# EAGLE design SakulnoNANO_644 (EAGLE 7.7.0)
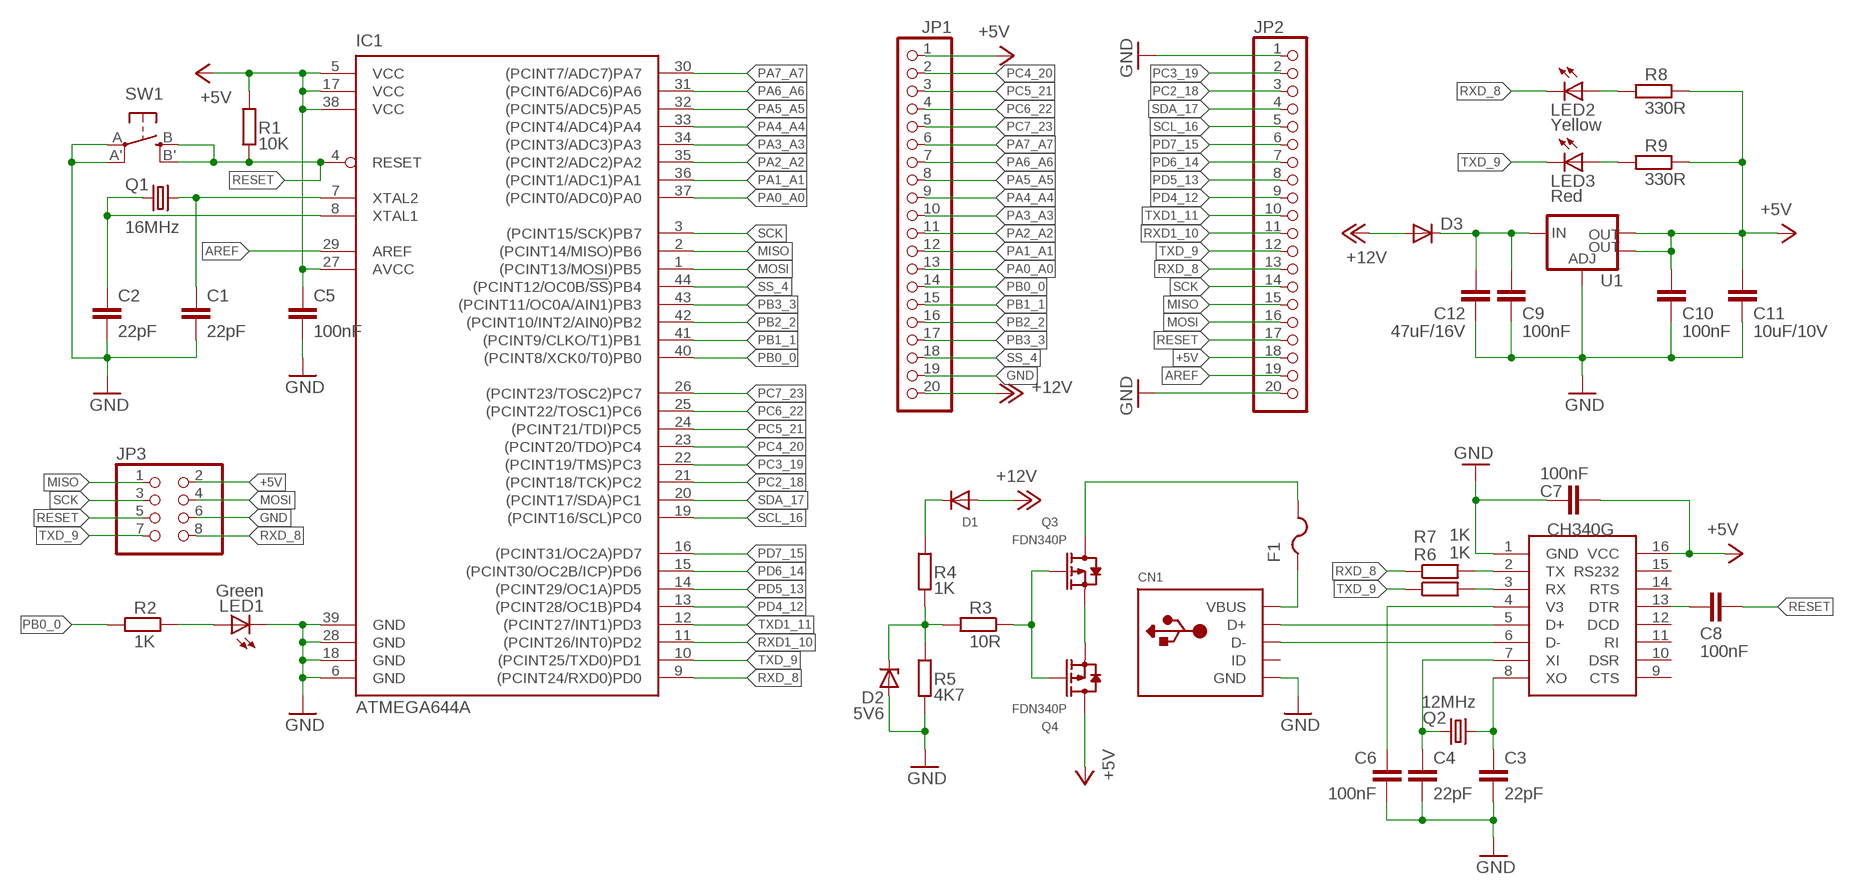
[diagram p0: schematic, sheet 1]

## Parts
C1  22pF  C-EUC1206  [C1206]
C2  22pF  C-EUC1206  [C1206]
C3  22pF  C-EUC1206  [C1206]
C4  22pF  C-EUC1206  [C1206]
C5  100nF  C-EUC1206  [C1206]
C6  100nF  C-EUC1206  [C1206]
C7  100nF  C-EUC1206  [C1206]
C8  100nF  C-EUC1206  [C1206]
C9  100nF  C-EUC1206  [C1206]
C10  100nF  C-EUC1206  [C1206]
C11  10uF/10V  C-EUC1206  [C1206]
C12  47uF/16V  C-EUC1206  [C1206]
CN1  USBMINIB  [USB-MINIB]
D1  DIODE_SOD-123FL  [SOD-123FL]
D2  5V6  ZENER-DIODESOD80C  [SOD80C]
D3  DIODE-DO214AC  [DO214AC]
F1  PTCFUSE-1206  [R1206]
IC1  ATMEGA644A  [TQFP44]
JP1  PINHD-1X20-BIG  [1X20-BIG]
JP2  PINHD-1X20-BIG  [1X20-BIG]
JP3  PINHD-2X4  [2X04]
LED1  Green  LEDCHIPLED_1206  [CHIPLED_1206]
LED2  Yellow  LEDCHIPLED_1206  [CHIPLED_1206]
LED3  Red  LEDCHIPLED_1206  [CHIPLED_1206]
Q1  16MHz  CRYSTALSM49  [SM49]
Q2  12MHz  CRYSTALSM49  [SM49]
Q3  FDN340P  SMD-MOSFET-P-CH-20V-2A-FDN340P(SOT-23)  [SOT-23]
Q4  FDN340P  SMD-MOSFET-P-CH-20V-2A-FDN340P(SOT-23)  [SOT-23]
R1  10K  R-EU_R1206  [R1206]
R2  1K  R-EU_R1206  [R1206]
R3  10R  R-EU_R1206  [R1206]
R4  1K  R-EU_R1206  [R1206]
R5  4K7  R-EU_R1206  [R1206]
R6  1K  R-EU_R1206  [R1206]
R7  1K  R-EU_R1206  [R1206]
R8  330R  R-EU_R1206  [R1206]
R9  330R  R-EU_R1206  [R1206]
SW1  SPST_TACT-EVQQ2  [EVQ-Q2]
U1  V_REG_LM1117SOT223  [SOT223]
U$1  CH340G  [SOIC16]

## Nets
+5V: C5.1 C7.2 C10.2 C11.2 IC1.5(VCC) IC1.17(VCC) IC1.27(AVCC) IC1.38(VCC) JP1.1 JP2.18 JP3.2 Q4.3(D) R1.2 R8.1 R9.1 U1.2(OUT) U1.4(OUT) U$1.16(VCC)
+12V: D1.A D3.A JP1.20
AREF: IC1.29(AREF) JP2.19
GND: C1.2 C2.2 C3.2 C4.2 C5.2 C6.2 C7.1 C9.1 C10.1 C11.1 C12.1 CN1.GND D2.A IC1.6(GND) IC1.18(GND) IC1.28(GND) IC1.39(GND) JP1.19 JP2.1 JP2.20 JP3.6 LED1.C R5.2 SW1.A'(P1) SW1.A(P) U1.1(ADJ) U$1.1(GND)
MISO: IC1.2((PCINT14/MISO)PB6) JP2.15 JP3.1
MOSI: IC1.1((PCINT13/MOSI)PB5) JP2.16 JP3.4
N$1: LED1.A R2.1
N$2: CN1.D+ U$1.5(D+)
N$3: C1.1 IC1.7(XTAL2) Q1.2
N$4: C2.1 IC1.8(XTAL1) Q1.1
N$5: CN1.D- U$1.6(D-)
N$6: CN1.VBUS F1.1
N$7: C4.1 Q2.1 U$1.7(XI)
N$8: C3.1 Q2.2 U$1.8(XO)
N$9: C8.1 U$1.13(DTR)
N$10: C6.1 U$1.4(V3)
N$11: R7.2 U$1.2(TX)
N$12: R6.2 U$1.3(RX)
N$13: Q3.2(S) Q4.2(S)
N$14: Q3.1(G) Q4.1(G) R3.1
N$15: D2.C R3.2 R4.2 R5.1
N$16: D1.C R4.1
N$17: LED2.A R8.2
N$18: LED3.A R9.2
N$22: C9.2 C12.2 D3.C U1.3(IN)
PA0_A0: IC1.37((PCINT0/ADC0)PA0) JP1.13
PA1_A1: IC1.36((PCINT1/ADC1)PA1) JP1.12
PA2_A2: IC1.35((PCINT2/ADC2)PA2) JP1.11
PA3_A3: IC1.34((PCINT3/ADC3)PA3) JP1.10
PA4_A4: IC1.33((PCINT4/ADC4)PA4) JP1.9
PA5_A5: IC1.32((PCINT5/ADC5)PA5) JP1.8
PA6_A6: IC1.31((PCINT6/ADC6)PA6) JP1.7
PA7_A7: IC1.30((PCINT7/ADC7)PA7) JP1.6
PB0_0: IC1.40((PCINT8/XCK0/T0)PB0) JP1.14 R2.2
PB1_1: IC1.41((PCINT9/CLKO/T1)PB1) JP1.15
PB2_2: IC1.42((PCINT10/INT2/AIN0)PB2) JP1.16
PB3_3: IC1.43((PCINT11/OC0A/AIN1)PB3) JP1.17
PC2_18: IC1.21((PCINT18/TCK)PC2) JP2.3
PC3_19: IC1.22((PCINT19/TMS)PC3) JP2.2
PC4_20: IC1.23((PCINT20/TDO)PC4) JP1.2
PC5_21: IC1.24((PCINT21/TDI)PC5) JP1.3
PC6_22: IC1.25((PCINT22/TOSC1)PC6) JP1.4
PC7_23: IC1.26((PCINT23/TOSC2)PC7) JP1.5
PD4_12: IC1.13((PCINT28/OC1B)PD4) JP2.9
PD5_13: IC1.14((PCINT29/OC1A)PD5) JP2.8
PD6_14: IC1.15((PCINT30/OC2B/ICP)PD6) JP2.7
PD7_15: IC1.16((PCINT31/OC2A)PD7) JP2.6
RESET: C8.2 IC1.4(RESET) JP2.17 JP3.5 R1.1 SW1.B'(S1) SW1.B(S)
RXD1_10: IC1.11((PCINT26/INT0)PD2) JP2.11
RXD_8: IC1.9((PCINT24/RXD0)PD0) JP2.13 JP3.8 LED2.C R7.1
SCK: IC1.3((PCINT15/SCK)PB7) JP2.14 JP3.3
SCL_16: IC1.19((PCINT16/SCL)PC0) JP2.5
SDA_17: IC1.20((PCINT17/SDA)PC1) JP2.4
SS_4: IC1.44((PCINT12/OC0B/!SS!)PB4) JP1.18
TXD1_11: IC1.12((PCINT27/INT1)PD3) JP2.10
TXD_9: IC1.10((PCINT25/TXD0)PD1) JP2.12 JP3.7 LED3.C R6.1
VBUS: F1.2 Q3.3(D)
Unconnected: CN1.ID U$1.9(CTS) U$1.10(DSR) U$1.11(RI) U$1.12(DCD) U$1.14(RTS) U$1.15(RS232)

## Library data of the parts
C1-C12 = rcl:C-EU: CAPACITOR, European symbol
CN1 = adafruit:USB: USB Connectors USBMINIB - Surface Mount Female Mini-B USB Connector 4UConnector: 06564 By microbuilder.eu Thru-hole RA Female Mini-B USB Connector 4UConnector: 18732 By ladyada.net
D1 = adafruit:DIODE: Diode
D2 = diode:ZENER-DIODE: Z-Diode
D3 = diode:DIODE-: DIODE
F1 = adafruit:PTCFUSE: PTC fuses, resettable thermistors
IC1 = atmel:ATMEGA644: 8-bit Microcontroller with 64K Bytes In-System Programmable Flash Source: http://www.atmel.com/dyn/resources/prod_documents/doc2593.pdf; MPN: ATMEGA644PV-10AU; OC_FARNELL: 1455123; OC_NEWARK: 58M3748
JP1 JP2 = adafruit:PINHD-1X20: PIN HEADER
JP3 = pinhead:PINHD-2X4: PIN HEADER
LED1-LED3 = adafruit:LED: LED
Q1 Q2 = crystal:CRYSTAL: CRYSTAL; OC_FARNELL: unknown; OC_NEWARK: unknown
Q3 Q4 = Seeed-Transistor:SMD-MOSFET-P-CH-20V-2A-FDN340P(SOT-23): 305030026; MPN: FDN340P
R1-R9 = rcl:R-EU_: RESISTOR, European symbol
SW1 = adafruit:SPST_TACT: SMT 6mm switch, EVQQ2 series http://www.ladyada.net/library/eagle
U1 = SparkFun-IC-Power:V_REG_LM1117: Voltage Regulator LM1117 Standard adjustable voltage regulator but in SMD form. Spark Fun Electronics SKU : COM-00595; PROD_ID: VREG-08170
U$1 = ch340g:CH340G

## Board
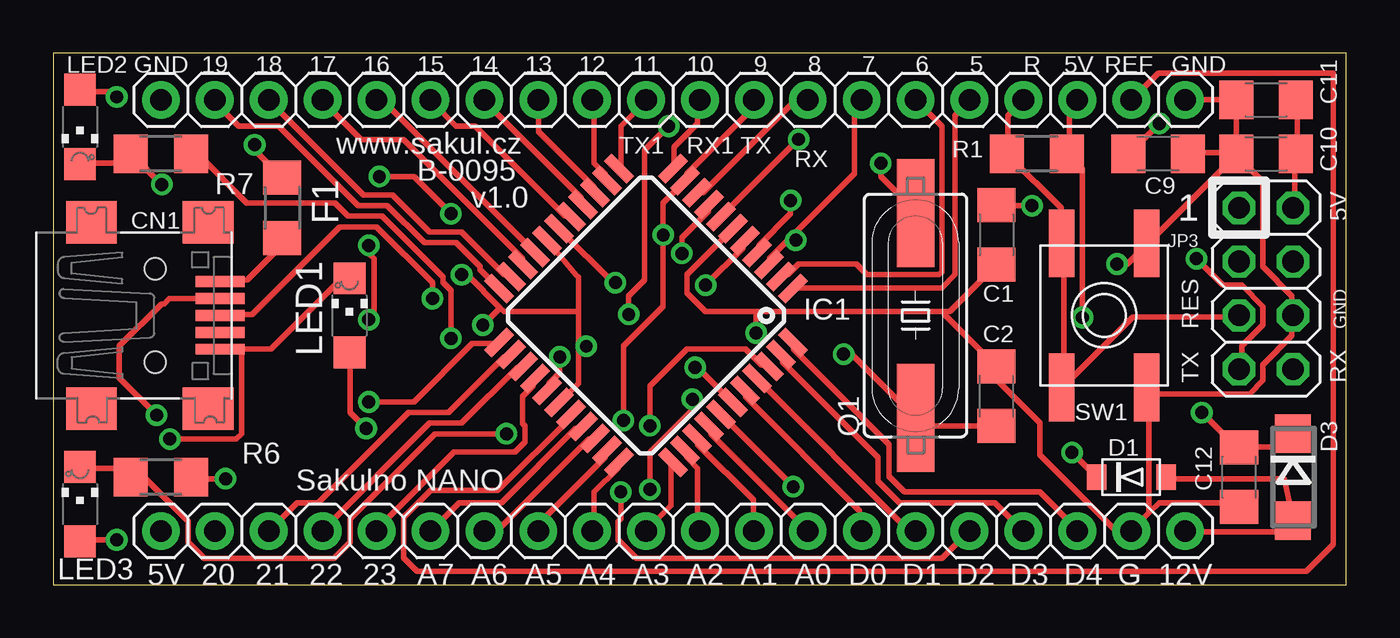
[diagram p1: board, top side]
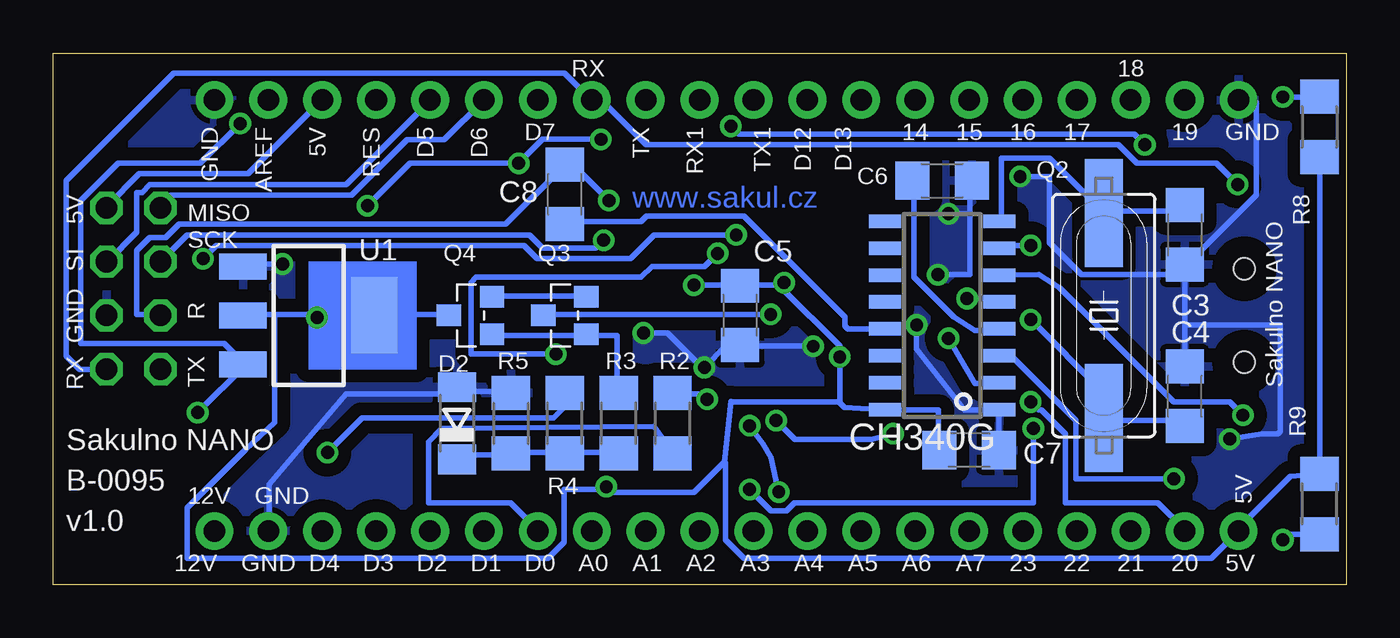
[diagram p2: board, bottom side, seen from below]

Size 60.94 x 25.07 mm. Coordinates in mm from the lower left corner, seen from the top.
Outline: 0,0 60.94,0 60.94,25.07 0,25.07 0,0
Copper layers (1*16): Top 0.035mm / dielectric 1.5mm / Bottom 0.035mm
Design rules "default": minimum track width 10mil, minimum drill 24mil, track to track 8mil, track to pad 8mil, pad to pad 8mil, via to via 8mil, smd to smd 8mil, copper to edge 40mil, drill to drill 8mil, minimum pad ring 10mil, minimum via ring 8mil, stop-mask expansion 4mil, vias tented up to drill 0mil, thermal gap 10mil

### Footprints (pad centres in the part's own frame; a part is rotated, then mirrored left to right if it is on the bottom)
C1206 = smd 1.6 x 1.8: 1 -1.4,0; 2 1.4,0
USB-MINIB = smd 0.5 x 2.308: D+ 0,4.064; D- -0.8,4.064; GND 1.6,4.064; ID 0.8,4.064; VBUS -1.6,4.064 | smd 2 x 2.4: GND1 -4.4,-2; GND2 -4.4,3.5; GND3 4.4,3.5; GND4 4.4,-2 | hole 1: -2.2,1; 2.2,1
SOD-123FL = smd 0.91 x 1.22: A 1.637,0; C -1.637,0
SOD80C = smd 1.4 x 1.8: A 1.7,0; C -1.7,0
DO214AC = smd 1.8 x 1.7: A 2.05,0; C -2.05,0
R1206 = smd 1.6 x 1.803: 1 -1.422,0; 2 1.422,0
TQFP44 = smd 1.5 x 0.5: 1 -5.8,4; 2 -5.8,3.2; 3 -5.8,2.4; 4 -5.8,1.6; 5 -5.8,0.8; 6 -5.8,0; 7 -5.8,-0.8; 8 -5.8,-1.6; 9 -5.8,-2.4; 10 -5.8,-3.2; 11 -5.8,-4; 23 5.8,-4; 24 5.8,-3.2; 25 5.8,-2.4; 26 5.8,-1.6; 27 5.8,-0.8; 28 5.8,0; 29 5.8,0.8; 30 5.8,1.6; 31 5.8,2.4; 32 5.8,3.2; 33 5.8,4 | smd 0.5 x 1.5: 12 -4,-5.8; 13 -3.2,-5.8; 14 -2.4,-5.8; 15 -1.6,-5.8; 16 -0.8,-5.8; 17 0,-5.8; 18 0.8,-5.8; 19 1.6,-5.8; 20 2.4,-5.8; 21 3.2,-5.8; 22 4,-5.8; 34 4,5.8; 35 3.2,5.8; 36 2.4,5.8; 37 1.6,5.8; 38 0.8,5.8; 39 0,5.8; 40 -0.8,5.8; 41 -1.6,5.8; 42 -2.4,5.8; 43 -3.2,5.8; 44 -4,5.8
1X20-BIG = drill 1.016 pad 1.778: 1 -24.13,0; 2 -21.59,0; 3 -19.05,0; 4 -16.51,0; 5 -13.97,0; 6 -11.43,0; 7 -8.89,0; 8 -6.35,0; 9 -3.81,0; 10 -1.27,0; 11 1.27,0; 12 3.81,0; 13 6.35,0; 14 8.89,0; 15 11.43,0; 16 13.97,0; 17 16.51,0; 18 19.05,0; 19 21.59,0; 20 24.13,0
2X04 = drill 1.016 octagon: 1 -3.81,-1.27; 2 -3.81,1.27; 3 -1.27,-1.27; 4 -1.27,1.27; 5 1.27,-1.27; 6 1.27,1.27; 7 3.81,-1.27; 8 3.81,1.27
CHIPLED_1206 = smd 1.5 x 1.5: A 0,-1.75; C 0,1.75
SM49 = smd 5.08 x 1.778: 1 -4.826,0; 2 4.826,0
SOT-23 = smd 1.016 x 1.143: 1 -0.889,-1.016; 2 0.889,-1.016; 3 0,1.016
EVQ-Q2 = smd 3.2 x 1.2: A -3.4,-2; A' 3.4,-2; B -3.4,2; B' 3.4,2
SOT223 = smd 1.219 x 2.235: 1 -2.311,-3.099; 2 0,-3.099; 3 2.311,-3.099 | smd 3.6 x 2.2: 4 0,3.099
SOIC16 = smd 0.635 x 1.524: 1 -4.445,-2.695; 2 -3.175,-2.695; 3 -1.905,-2.695; 4 -0.635,-2.695; 5 0.635,-2.695; 6 1.905,-2.695; 7 3.175,-2.695; 8 4.445,-2.695; 9 4.445,2.695; 10 3.175,2.695; 11 1.905,2.695; 12 0.635,2.695; 13 -0.635,2.695; 14 -1.905,2.695; 15 -3.175,2.695; 16 -4.445,2.695

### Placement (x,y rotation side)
C1  44.45,16.51 270 top
C2  44.45,8.89 90 top
C3  7.62,16.51 270 bottom
C4  7.62,8.89 90 bottom
C5  28.57,12.7 270 bottom
C6  19.05,19.05 0 bottom
C7  17.78,6.35 180 bottom
C8  36.83,18.41 90 bottom
C9  52.07,20.32 180 top
C10  57.15,20.32 0 top
C11  57.15,22.86 0 top
C12  55.88,5.08 90 top
CN1  3.81,12.7 270 top
D1  50.8,5.08 0 top
D2  41.91,7.62 90 bottom
D3  58.42,5.08 270 top
F1  10.79,17.78 90 top
IC1  27.94,12.7 225 top
JP1  29.21,2.54 0 top
JP2  29.21,22.86 0 top
JP3  57.15,13.97 270 top
LED1  13.97,12.7 0 top
LED2  1.27,21.59 180 top
LED3  1.27,3.81 0 top
Q1  40.64,12.7 90 top
Q2  11.43,12.7 90 bottom
Q3  36.83,12.7 90 bottom
Q4  41.27,12.7 90 bottom
R1  46.35,20.32 0 top
R2  31.75,7.62 270 bottom
R3  34.29,7.62 270 bottom
R4  36.83,7.62 270 bottom
R5  39.37,7.62 90 bottom
R6  5.08,5.08 0 top
R7  5.08,20.32 0 top
R8  1.27,21.59 90 bottom
R9  1.27,3.81 270 bottom
SW1  49.53,12.7 90 top
U1  48.9,12.7 270 bottom
U$1  19.05,12.7 90 bottom

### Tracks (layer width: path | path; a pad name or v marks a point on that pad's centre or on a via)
+5V  (via drill 0.61)
  Top 0.254: JP2.18 48.25,22.75 47.88,22.38 47.88,20.38 R1.2 47.88,20.25 48.5,19.62 v48.5,12.61 | C11.2 58.62,22.75 58.62,20.38 C10.2 58.5,20.25 58.5,17.88 JP3.2 | v26.5,14.25 26.38,14.25 23.88,16.75 IC1.17 | v30.75,14.12 32.5,15.88 32.5,16.12 IC1.5 | v34.88,4.62 31.5,8 IC1.38 | v23.88,10.75 23.88,10 23.38,9.5 23.38,9.25 IC1.27
  Bottom 0.254: Q4.3 42.38,12.75 45.75,12.75 U1.4 45.88,12.75 48.5,12.75 | 48.5,12.75 50.5,12.75 | 50.5,12.75 51.88,12.75 U1.2 | JP2.18 48.38,22.75 51.75,19.38 56.88,19.38 58.38,17.88 JP3.2 | v48.5,12.61 48.5,12.75 | R8.1 1.25,20.12 1.25,5.25 R9.1 2.65,5.12 5.14,2.62 5,2.62 JP1.1 5.12,2.5 6.38,1.25 28.38,1.25 29.25,2.12 29.25,5.74 29.31,5.8 | v30.75,14.12 28.62,14.12 C5.1 28.5,14.12 26.62,14.12 v26.5,14.25 26.62,14 23.88,11.25 v23.88,10.75 23.88,8.62 23.91,8.62 | 29.31,5.8 29,8.65 29,8.62 23.91,8.62 | 29.31,5.8 30.75,4.37 34.5,4.37 v34.88,4.62 34.88,4.5 36.88,4.5 36.88,2 37.62,1.25 54.62,1.25 54.62,3.63 51.88,6.38 50.5,7.66 50.5,12.75 | 23.91,8.62 23.66,8.38 U$1.16 21.62,8.25 19.23,8.25 19.23,6.38 C7.2
+12V
  Top 0.254: D1.A 52.5,5 58.02,5 58.38,3.38 58.38,3.12 D3.A 58.25,3.12 57.62,2.5 53.38,2.5 JP1.20
AREF
  Top 0.254: IC1.29 24.4,7.89 20.95,4.45 17.78,4.45 16.51,3.17 16.51,1.27 17.14,0.64 59.05,0.64 60.33,1.91 60.33,24.13 52.07,24.13 JP2.19
GND  (via drill 0.61)
  Top 0.254: LED1.C 13.88,14.38 13.52,14.38 10.27,11.12 7.88,11.12 CN1.GND 8.88,11 8.88,7.12 8.62,6.88 v5.5,6.88 | v30.25,10.25 30.38,10.25 32,8.62 IC1.39 | 24.75,11.25 24.75,9.5 23.88,8.62 IC1.28 | 24.75,11.25 24.75,12.88 | 24.75,12.88 24.75,14.5 24.64,14.61 23.38,16.12 IC1.18 | v19.25,14.62 19.5,14.62 21.06,13.06 | 21.06,13.06 21.25,12.88 24.75,12.88 | 21.06,13.06 v20.25,12.25 | 24.75,11.25 v25.12,11.25 | v15.38,19.25 17,19.25 v18.75,17.5 | v50.12,15.12 50.62,15.12 51.5,16 SW1.A' 51.62,16.12 55.75,20.25 | C9.1 53.5,20.38 55.75,20.38 C10.1 | C10.1 C11.1 55.62,22.88 53.38,22.88 JP2.20 | 55.75,20.25 57,19 57,15 58.38,13.62 58.38,12.75 JP3.6 58.38,12.62 58.38,11.75 57,10.38 57,9.62 56.38,9 51.75,9 SW1.A 51.62,9.25 51.62,3.5 51.69,3.44 | 55.75,20.25 C10.1 | 42,12.88 42.25,12.88 44.38,15 C1.2 | 42,12.88 33.12,12.88 | 33.12,12.88 30.75,12.88 29.88,13.75 29.88,14.62 32,16.75 IC1.6 | 42,12.88 42,12.75 44.38,10.38 C2.2 44.5,10.25 44.5,9.62 46.5,7.62 46.5,6.12 50,2.62 50.75,2.62 JP1.19 50.88,2.62 51.69,3.44 | 51.69,3.44 52.12,3.88 55.66,3.88 55.78,3.75 55.88,3.75 C12.1 | 33.12,12.88 v33.12,11.88
  Bottom 0.254: 7.62,12.25 7.62,15 C3.2 | 7.62,12.25 7.62,10.38 C4.2 | C3.2 7.5,15.12 4.25,18.38 4.25,22.75 5,22.75 JP2.1 | v5.5,6.88 3.98,7.12 3.23,7.12 3.12,7.23 3.12,12.25 7.62,12.25 | C7.1 16.36,6.38 16.38,6.38 16.38,8.25 U$1.1 16.5,8.25 17.12,8.24 18.01,8.24 20.25,11.12 v20.25,12.25 | 17.75,17.5 17.75,14.62 v19.25,14.62 | 17.75,17.5 17.75,19 C6.2 | v25.12,11.25 28.5,11.25 C5.2 28.62,11.25 29.25,11.25 v30.25,10.25 30.38,10.25 32,11.88 v33.12,11.88 | v15.38,19.25 14,19.25 14,16.12 12.5,14.62 7.75,14.62 C3.2 | 17.75,17.5 v18.75,17.5 | v50.12,15.12 51.88,15.12 U1.1 | R5.2 39.38,9.12 41.75,9.12 41.88,9.25 D2.A 42,9.25 42.88,9.01 47.12,9.01 50.75,4.75 50.75,2.62 JP1.19
  pour Bottom (isolate 0.61): 0,24.77 60.96,24.77 60.96,0 0,0
MISO
  Top 0.254: JP2.15 41.88,21.62 41.88,14.75 41.75,14.62 38.35,14.62 37.85,15.12 35.12,15.12 34.62,14.62 34.38,14.62 IC1.2
  Bottom 0.254: JP2.15 42.51,20.99 44.26,20.99 46.88,18.38 55.38,18.38 55.88,17.88 JP3.1
MOSI
  Top 0.254: IC1.1 34.88,14 41.88,14 42.5,14.62 42.5,22.12 43.12,22.75 JP2.16
  Bottom 0.254: JP3.4 58.38,15.25 57,16.62 57,18.5 56.75,18.5 56.38,18.88 47.12,18.88 43.25,22.75 JP2.16
N$1  (via drill 0.61)
  Top 0.254: v14.75,7.38 14,8.12 14,10.88 LED1.A | v28.12,4.5 28.12,6.25 30.12,8.25 v30.12,8.75
  Bottom 0.254: v14.75,7.38 14.75,3.88 26,3.88 26.38,3.5 27.12,3.5 v28.12,4.5 | v30.12,8.75 30.38,9 31.75,9 R2.1
N$2  (via drill 0.61)
  Top 0.254: v17.88,13.5 17.88,14.25 15.25,16.88 13.5,16.88 9.38,12.75 7.88,12.75 CN1.D+
  Bottom 0.254: v17.88,13.5 16.5,13.5 16.38,13.38 U$1.5
N$3  (via drill 0.61)
  Top 0.254: v35.12,21 31.5,17.38 IC1.7 | v39,19.88 39,19.25 40.62,17.62 Q1.2 | v46.12,17.88 44.5,17.88 C1.1
  Bottom 0.254: v35.12,21 37.88,21 v39,19.88 44.12,19.88 v46.12,17.88
N$4  (via drill 0.61)
  Top 0.254: v29.62,15.62 29.62,16.38 30.88,17.62 30.88,17.88 IC1.8 | v37.25,10.88 37.62,10.88 40.62,7.88 Q1.1 40.75,7.75 41,7.5 44.38,7.5 C2.1
  Bottom 0.254: v29.62,15.62 30.25,15 32.73,15 33.23,14.5 41,14.5 41.25,14.25 41.25,10.88 v37.25,10.88
N$5  (via drill 0.61)
  Top 0.254: v4.88,8 3.12,9.75 3.12,11.25 5.12,13.25 5.23,13.25 5.48,13.5 CN1.D-
  Bottom 0.254: U$1.6 14.48,14.63 13.5,14 8.12,8.62 5.5,8.62 v4.88,8
N$6
  Top 0.254: F1.1 10.75,16.25 11.02,16.25 9.14,14.38 CN1.VBUS
N$7  (via drill 0.61)
  Top 0.254: v14.88,16 14.88,15.62 15.12,15.38 15.12,12.75 v14.88,12.5
  Bottom 0.254: v14.88,16 16.12,16 16.25,15.88 U$1.7 | v14.88,12.5 11.5,9.12 11.5,7.88 Q2.1 11.38,7.75 7.88,7.75 C4.1
N$8
  Bottom 0.254: U$1.8 16.25,17.25 16.25,20.12 14,20.12 11.5,17.62 Q2.2 11.38,17.62 7.88,17.62 7.62,17.88 C3.1
N$9
  Bottom 0.254: C8.1 36.75,17.12 33.23,17.12 32.98,17.38 28.38,17.38 23.62,12.62 23.62,12.2 23.5,12.06 U$1.13
N$10
  Bottom 0.254: C6.1 20.38,19 20.38,14.5 18.5,12.62 17.51,11.99 16.43,11.99 U$1.4
N$11  (via drill 0.61)
  Top 0.254: v18.75,11.62 18.75,13.88 18.38,14.25 18.38,14.5 15.5,17.38 13.9,17.38 13.28,18 9.12,18 6.88,20.25 6.62,20.25 R7.2
  Bottom 0.254: v18.75,11.62 17.89,10.12 17.51,9.49 16.39,9.49 U$1.2 17.01,9.62
N$12  (via drill 0.61)
  Top 0.254: v8.12,5 6.62,5 R6.2
  Bottom 0.254: v8.12,5 12.75,5 12.75,7.75 15.88,10.88 16.39,10.88 16.25,10.75 U$1.3
N$13
  Bottom 0.254: Q3.2 35.88,13.62 40.25,13.62 Q4.2
N$14
  Bottom 0.254: Q4.1 40.25,11.75 35.88,11.75 Q3.1 35.75,11.75 34.38,11.75 34.38,9.12 R3.1
N$15
  Bottom 0.254: R3.2 34.38,6.25 36.75,6.25 R4.2 36.88,6.25 39.25,6.25 R5.1 39.38,6.12 41.75,6.12 41.88,6 D2.C
N$16  (via drill 0.61)
  Top 0.254: v48.01,6.24 49.12,5.12 D1.C
  Bottom 0.254: v48.01,6.24 46.38,7.88 37.37,7.88 36.24,9 R4.1
N$17  (via drill 0.61)
  Top 0.254: v3,23 2.75,23.25 1.38,23.25 LED2.A
  Bottom 0.254: v3,23 1.38,23 R8.2
N$18  (via drill 0.61)
  Top 0.254: v3,2.12 1.38,2.12 LED3.A
  Bottom 0.254: v3,2.12 2.75,2.38 1.38,2.38 R9.2
N$22  (via drill 0.61)
  Top 0.254: D3.C 58.38,7.12 57.75,6.5 56,6.5 C12.2 55.75,6.5 v54.12,8.12 | v52.12,21.75 50.75,20.38 C9.2
  Bottom 0.254: v52.12,21.75 54,19.88 57.88,19.88 59.62,18.12 59.62,11.38 52.88,11.38 52,10.5 U1.3 51.88,10.38 v54.12,8.12
PA0_A0
  Top 0.254: IC1.37 31,7.38 31,7.12 35.5,2.62 JP1.13
PA1_A1
  Top 0.254: IC1.36 30.38,6.88 30.38,6.62 33,4 33,2.62 JP1.12
PA2_A2
  Top 0.254: IC1.35 29.88,6.25 29.88,6 30.38,5.5 30.38,2.62 JP1.11
PA3_A3
  Top 0.254: IC1.34 29.12,5.75 29.12,3.75 28,2.62 JP1.10
PA4_A4
  Top 0.254: IC1.33 26.62,5.75 26.62,5.5 25.5,4.38 25.5,2.62 JP1.9
PA5_A5
  Top 0.254: IC1.32 26,6.25 26,6 22.88,2.88 22.88,2.62 JP1.8
PA6_A6
  Top 0.254: IC1.31 25.5,6.88 25.25,6.88 21,2.62 20.38,2.62 JP1.7
PA7_A7
  Top 0.254: IC1.30 24.88,7.38 24.62,7.38 21.12,3.88 19.12,3.88 17.88,2.62 JP1.6
PB0_0
  Top 0.254: IC1.40 32.62,9.12 32.62,8.88 38,3.5 38,2.62 JP1.14
  Bottom 0.254: R2.2 31.75,6.25 32.63,7.47 42.62,7.38 43.25,6.75 43.25,3.88 39.38,3.88 38.12,2.62 JP1.14
PB1_1
  Top 0.254: IC1.41 33.25,9.62 40.25,2.62 40.62,2.62 JP1.15
PB2_2  (via drill 0.61)
  Top 0.254: v28.12,7.5 28.12,9.38 29.88,11.12 32.62,11.12 33.38,10.38 33.62,10.38 IC1.42 | v26.75,4.38 26.75,3.12 26.62,3 26.62,2.12 27.5,1.25 41.88,1.25 43.12,2.5 JP1.16
  Bottom 0.254: v28.12,7.5 27.49,6.64 27.11,6.01 v26.75,4.38
PB3_3
  Top 0.254: IC1.43 34.38,10.75 34.38,10.5 38.88,6 38.88,4.88 39.88,3.88 44.38,3.88 45.62,2.62 JP1.17
PC2_18
  Top 0.254: IC1.21 21.5,14.62 21.25,14.62 19.25,16.62 17.75,16.62 16,18.38 14.62,18.38 10.25,22.75 JP2.3
PC3_19
  Top 0.254: IC1.22 21,14 20.12,14.88 20.12,15 19,16.12 17.5,16.12 15.75,17.88 14.38,17.88 10.62,21.62 8.75,21.62 7.62,22.75 JP2.2
PC4_20  (via drill 0.61)
  Top 0.254: v14.88,8.62 17,8.62 19.75,11.38 21,11.38 IC1.23
  Bottom 0.254: v14.88,8.62 14.5,8.25 14.38,8.25 13.25,7.12 13.25,3.88 8.88,3.88 7.62,2.62 JP1.2
PC5_21
  Top 0.254: IC1.24 21.5,10.75 21.25,10.75 18.62,8.12 16.75,8.12 12.5,3.88 11.5,3.88 10.25,2.62 JP1.3
PC6_22
  Top 0.254: IC1.25 22.12,10.25 21.88,10.25 19.25,7.62 17.75,7.62 12.75,2.62 JP1.4
PC7_23
  Top 0.254: IC1.26 22.62,9.62 22.62,9.38 22.12,8.88 22.12,7.62 22.24,7.5 22.24,6.75 21.77,6.28 18.91,6.28 15.25,2.62 JP1.5
PD4_12
  Top 0.254: IC1.13 26,19.12 26,19.38 25.5,19.88 25.5,22.75 JP2.9
PD5_13
  Top 0.254: IC1.14 25.5,18.5 25.5,18.75 22.88,21.38 22.88,22.75 JP2.8
PD6_14
  Top 0.254: IC1.15 24.88,18 24.88,18.25 20.38,22.75 JP2.7
PD7_15
  Top 0.254: IC1.16 24.38,17.38 24.12,17.38 19.88,21.62 19,21.62 17.88,22.75 JP2.6
RESET  (via drill 0.61)
  Top 0.254: v34.75,18.12 34.75,17.5 33.25,16 33.25,15.75 IC1.4 | JP2.17 45.62,22.75 45,22.12 45,20.38 R1.1 45,20.25 47.5,17.75 47.5,16.12 SW1.B' 47.62,16 47.62,9.5 SW1.B 47.62,9.38 50.88,12.62 55.88,12.62 JP3.5
  Bottom 0.254: v34.75,18.12 36.38,19.75 36.75,19.75 C8.2 36.88,19.75 39.62,17 55,17 55.62,16.38 56.38,16.38 57,15.75 57,12.75 56,12.75 JP3.5
RXD1_10
  Top 0.254: IC1.11 29.25,19.75 29.25,20.62 30.38,21.75 30.38,22.75 JP2.11
RXD_8  (via drill 0.61)
  Top 0.254: LED2.C 1.38,19.88 3.25,19.88 3.62,20.25 R7.1 3.75,20.25 v5.12,18.88 | IC1.9 30.38,18.5 30.62,18.5 34.88,22.75 35.5,22.75 JP2.13
  Bottom 0.254: v5.12,18.88 6.12,19.88 9.88,19.88 10.75,20.75 33,20.75 35,22.75 35.5,22.75 JP2.13 36.83,24.13 55.24,24.13 60.33,19.05 60.33,10.79 59.69,10.16 JP3.8
  Bottom 0.406: 35.5,22.75 35.5,22.8
SCK  (via drill 0.61)
  Top 0.254: 34.81,16.44 37.75,19.38 37.75,22.5 38,22.75 JP2.14 | 34.81,16.44 33.75,15.38 33.75,15.12 IC1.3 | 34.81,16.44 v35,16.25
  Bottom 0.254: v35,16.25 35.38,15.88 37.88,15.88 38.5,16.5 54.62,16.5 JP3.3
SCL_16
  Top 0.254: IC1.19 22.62,15.75 15.62,22.75 15.25,22.75 JP2.5
SDA_17
  Top 0.254: IC1.20 22.12,15.12 22.12,15.38 16.51,20.99 14.51,20.99 12.75,22.75 JP2.4
SS_4
  Top 0.254: IC1.44 34.88,11.38 34.88,11.12 39.38,6.62 39.38,5.12 40.12,4.38 46.5,4.38 48.25,2.62 JP1.18
TXD1_11
  Top 0.254: IC1.12 26.75,19.75 26.75,21.62 27.88,22.75 JP2.10
TXD_9  (via drill 0.61)
  Top 0.254: LED3.C 1.38,5.5 3.25,5.5 3.62,5.12 R6.1 3.75,5 4.38,5 6.38,3 6.38,2 7.12,1.25 13.25,1.25 14,2 14,3.12 18,7.12 v21.36,7.12 | JP2.12 33,22.75 33,22.5 29.88,19.38 29.88,19.12 IC1.10 29.75,19 28.75,18 v28.75,16.5 28.75,13.12 26.88,11.25 v26.88,7.75 | v53.88,15.38 55.12,14.12 56,14.12 57,13.12 57,12.25 56,11.25 56,10.25 JP3.7
  Bottom 0.254: v21.36,7.12 22.38,6.87 25.99,6.87 v26.88,7.75 | v53.88,15.38 53.25,16 38.75,16 38.12,15.38 33.74,15.38 32.62,16.5 v28.75,16.5
VBUS  (via drill 0.61)
  Top 0.254: v27.12,12.75 27.12,13.62 27.88,14.38 27.88,20.5 v29,21.62 | v9.5,20.75 9.5,20.5 10.75,19.25 F1.2
  Bottom 0.254: v27.12,12.75 37.75,12.75 Q3.3 | v29,21.62 28.62,21.25 10,21.25 v9.5,20.75
(copper drawn outside any net)
  shapes: Bottom area x1

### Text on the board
Bottom: www.sakul.cz
tPlace: GND | 19 | 18 | 17 | 16 | 15 | 14 | 13 | 12 | 11 | 10 | 9 | 8 | 7 | 6 | 5 | R | 5V | REF | GND | www.sakul.cz | TX1 | RX1 | TX | RX | B-0095 | v1.0 | 1 | 5V | RES | GND | TX | RX | Sakulno NANO | 5V | 20 | 21 | 22 | 23 | A7 | A6 | A5 | A4 | A3 | A2 | A1 | A0 | D0 | D1 | D2 | D3 | D4 | G | 12V
bPlace: 18 | RX | D13 | D12 | TX1 | RX1 | TX | D6 | D5 | RES | 5V | AREF | GND | GND | 19 | 17 | 16 | 15 | 14 | D7 | 5V | Sakulno NANO | MISO | SCK | SI | GND | R | TX | RX | Sakulno NANO | 5V | GND | 12V | B-0095 | v1.0 | 5V | 20 | 21 | 22 | 23 | A7 | A6 | A5 | A4 | A3 | A2 | A1 | A0 | D0 | D1 | D2 | D3 | D4 | GND | 12V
